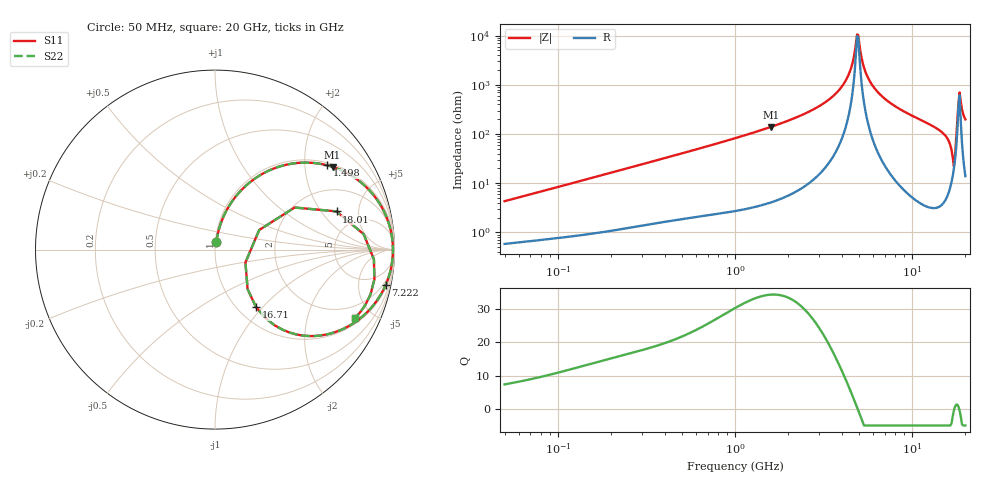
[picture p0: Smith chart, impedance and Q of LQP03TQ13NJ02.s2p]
!Murata Part Number: LQP03TQ13NJ02
!These Parameters are Measured in Series Mode Connection
!  o--[Z]--o
!Port1  Port2
!  o-------o
!Freq. Start=50[MHz] Stop=20[GHz], 401[Steps]
# Hz S RI R 50
!Freq.(Hz) S11(Real) S11(Imag) S21(Real) S21(Imag) S12(Real) S12(Imag) S22(Real) S22(Imag)
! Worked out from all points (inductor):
!   401 points, 50 MHz to 20 GHz, reference 50 ohm
!   read as one part in series: L = 13.5 nH near 51.52 MHz
!   highest Q = 34.3 at 1.591 GHz (marker M1), where L = 13.9 nH
!   self-resonance near 4.893 GHz
!   S11 on the Smith chart (normalised r, x): 50 MHz: 1.01, +0.09; 1.498 GHz: 1.08, +2.59; 7.222 GHz: 1.38, -9.56; 16.71 GHz: 1.21, -0.92; 18.01 GHz: 3.32, +2.85; 20 GHz: 1.28, -3.95
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5e7  0.00759 0.0422  0.9924 -0.0422  0.9924 -0.0422  0.00759 0.0422
1.364002e8  0.021 0.1094  0.979 -0.1094  0.979 -0.1094  0.021 0.1094
3.721004e8  0.0947 0.2679  0.9053 -0.2679  0.9053 -0.2679  0.0947 0.2679
1e9  0.4056 0.4748  0.5944 -0.4748  0.5944 -0.4748  0.4056 0.4748
1.498439e9  0.6227 0.4703  0.3773 -0.4703  0.3773 -0.4703  0.6227 0.4703
1.590961e9  0.6551 0.461  0.3449 -0.461  0.3449 -0.461  0.6551 0.461
2.728004e9  0.8955 0.2881  0.1045 -0.2881  0.1045 -0.2881  0.8955 0.2881
4.087748e9  0.9815 0.0953  0.0185 -0.0953  0.0185 -0.0953  0.9815 0.0953
4.472136e9  0.9885 0.0496  0.0115 -0.0496  0.0115 -0.0496  0.9885 0.0496
4.89267e9  0.9913 0.00345  0.00873 -0.00345  0.00873 -0.00345  0.9913 0.00345
5.041459e9  0.9912 -0.012  0.00879 0.012  0.00879 0.012  0.9912 -0.012
5.352748e9  0.9896 -0.043  0.0104 0.043  0.0104 0.043  0.9896 -0.043
5.683258e9  0.986 -0.074  0.014 0.074  0.014 0.074  0.986 -0.074
7.222371e9  0.9509 -0.197  0.0491 0.197  0.0491 0.197  0.9509 -0.197
7.442007e9  0.944 -0.2121  0.056 0.2121  0.056 0.2121  0.944 -0.2121
1.438523e10  0.5747 -0.48  0.4253 0.48  0.4253 0.48  0.5747 -0.48
1.597544e10  0.3782 -0.4472  0.6218 0.4472  0.6218 0.4472  0.3782 -0.4472
1.670968e10  0.2287 -0.3201  0.7713 0.3201  0.7713 0.3201  0.2287 -0.3201
1.721783e10  0.1695 -0.0717  0.8305 0.0717  0.8305 0.0717  0.1695 -0.0717
1.800918e10  0.6771 0.2128  0.3229 -0.2128  0.3229 -0.2128  0.6771 0.2128
1.88369e10  0.8879 -0.1662  0.1121 0.1662  0.1121 0.1662  0.8879 -0.1662
2e10  0.7812 -0.3798  0.2188 0.3798  0.2188 0.3798  0.7812 -0.3798
